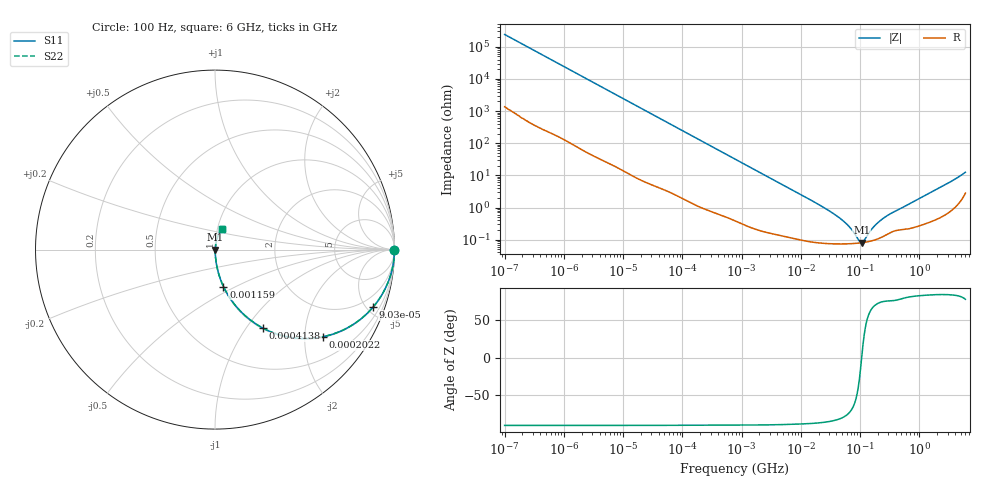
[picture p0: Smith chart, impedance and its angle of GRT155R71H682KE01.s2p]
!Murata Part Number: GRT155R71H682KE01
!These Parameters are Measured in Series Mode Connection
!Data Generated on Jun 19, 2026
!  o--ll--o
!Port1  Port2
!  o------o
!Operation Temp=25[degC], DC Bias Voltage=0[V]
!Freq. Start=100[Hz] Stop=6[GHz] 401[Steps]
# Hz S RI R 50
!Freq.(Hz) S11(Real) S11(Imag) S21(Real) S21(Imag) S12(Real) S12(Imag) S22(Real) S22(Imag)
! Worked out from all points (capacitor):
!   401 points, 100 Hz to 6 GHz, reference 50 ohm
!   read as one part in series: C = 6.57 nF near 109 Hz
!   lowest |Z| = 79.9 mohm at 106.7 MHz (marker M1)
!   series resonance near 106.4 MHz, so ESL is about 340 pH
!   S11 on the Smith chart (normalised r, x): 100 Hz: open; 90.3 kHz: 1.04, -5.49; 202.2 kHz: 1.02, -2.46; 413.8 kHz: 1.01, -1.21; 1.159 MHz: 1.01, -0.43; 6 GHz: 1.06, +0.24
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100  1 -0.000413  2.5e-06 0.000413  2.5e-06 0.000413  1 -0.000413
2008  0.9999 -0.00822  0.00011 0.00822  0.00011 0.00822  0.9999 -0.00822
12592  0.9971 -0.0511  0.0029 0.0511  0.0029 0.0511  0.9971 -0.0511
40335  0.973 -0.1588  0.027 0.1588  0.027 0.1588  0.973 -0.1588
90302  0.8809 -0.3201  0.1191 0.3201  0.1191 0.3201  0.8809 -0.3201
135116  0.7697 -0.4171  0.2303 0.4171  0.2303 0.4171  0.7697 -0.4171
202169  0.6013 -0.4855  0.3987 0.4855  0.3987 0.4855  0.6013 -0.4855
289253  0.4264 -0.4901  0.5736 0.4901  0.5736 0.4901  0.4264 -0.4901
413847  0.2688 -0.4383  0.7312 0.4383  0.7312 0.4383  0.2688 -0.4383
774597  0.0976 -0.2909  0.9024 0.2909  0.9024 0.2909  0.0976 -0.2909
1159002  0.0473 -0.206  0.9527 0.206  0.9527 0.206  0.0473 -0.206
3394479  0.00698 -0.0738  0.993 0.0738  0.993 0.0738  0.00698 -0.0738
1.555665e7  0.0011 -0.0161  0.9989 0.0161  0.9989 0.0161  0.0011 -0.0161
4.983056e7  0.000752 -0.00402  0.9992 0.00402  0.9992 0.00402  0.000752 -0.00402
6.817316e7  0.000751 -0.00222  0.9992 0.00222  0.9992 0.00222  0.000751 -0.00222
9.753859e7  0.000784 -0.000421  0.9992 0.000421  0.9992 0.000421  0.000784 -0.000421
1.066761e8  0.000799 1.07e-05  0.9992 -1.07e-05  0.9992 -1.07e-05  0.000799 1.07e-05
1.166697e8  0.000818 0.000442  0.9992 -0.000442  0.9992 -0.000442  0.000818 0.000442
1.825626e8  0.001 0.0027  0.999 -0.0027  0.999 -0.0027  0.001 0.0027
3.124326e8  0.00162 0.0059  0.9984 -0.0059  0.9984 -0.0059  0.00162 0.0059
1.95892e9  0.00554 0.0359  0.9945 -0.0359  0.9945 -0.0359  0.00554 0.0359
6e9  0.0406 0.1138  0.9594 -0.1138  0.9594 -0.1138  0.0406 0.1138
